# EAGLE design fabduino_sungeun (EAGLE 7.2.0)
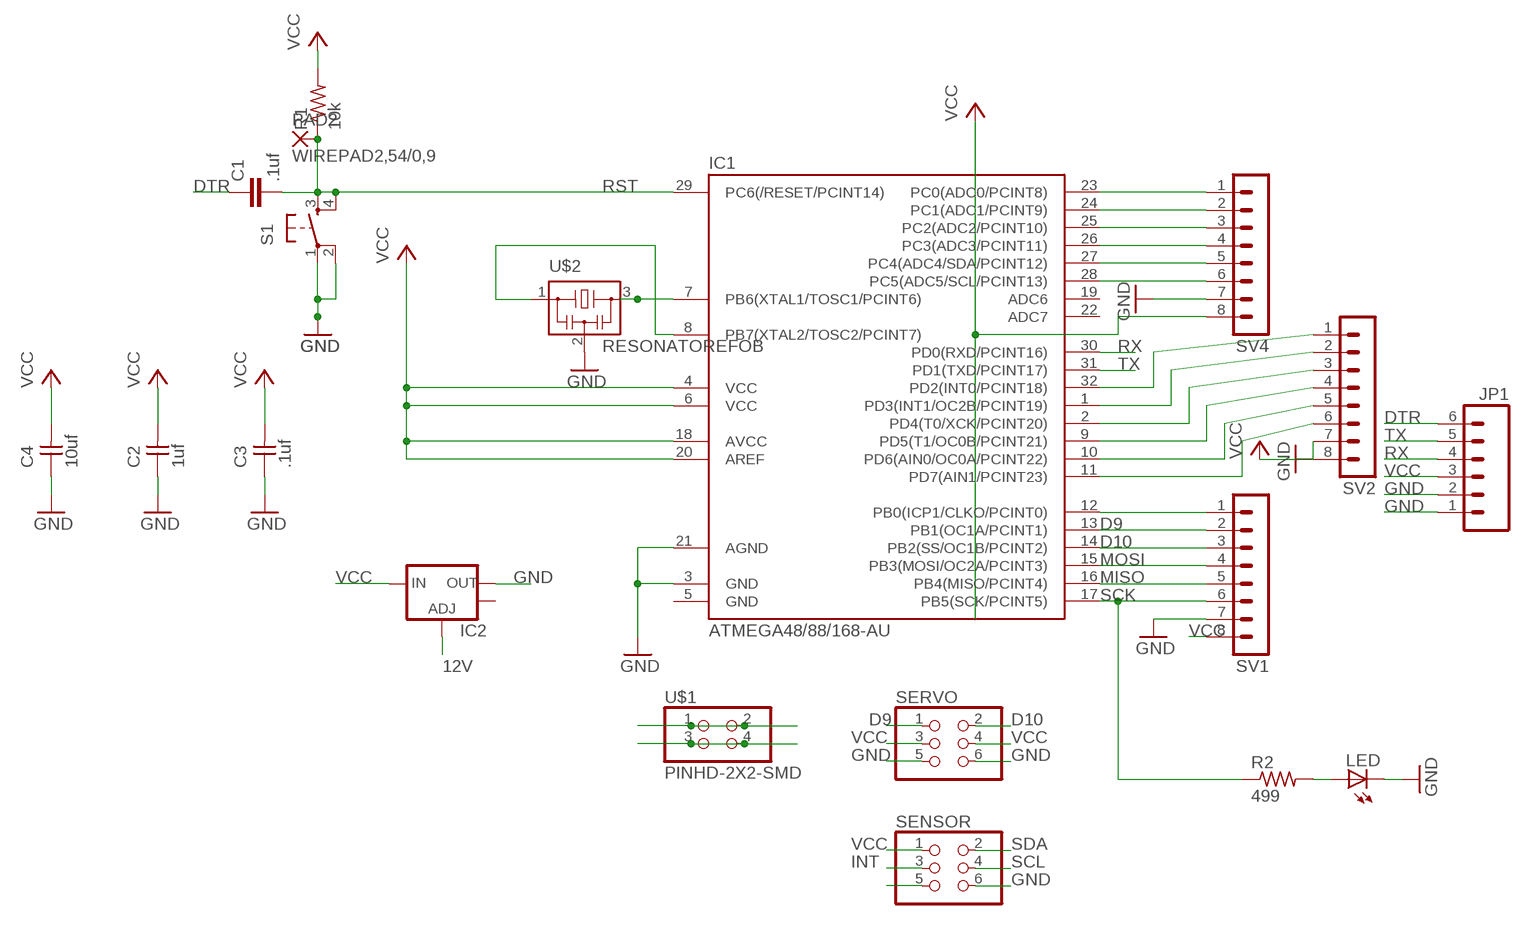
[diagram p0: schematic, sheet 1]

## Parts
C1  .1uf  C-EUC1206  [C1206]
C2  1uf  UNPOLARIZED_CAPACITOR1206  [1206]
C3  .1uf  UNPOLARIZED_CAPACITOR1206  [1206]
C4  10uf  UNPOLARIZED_CAPACITOR1206  [1206]
IC1  ATMEGA48/88/168-AU  [TQFP32-08]
IC2  V_REG_LM1117SOT223  [SOT223]
JP1  M06SMD  [1X06-SMD]
LED  LED1206  [1206]
PAD2  WIREPAD2,54/0,9  [2,54/0,9]
R1  10k  RESISTOR1206  [1206]
R2  499  RESISTOR1206  [1206]
S1  6MM_SWITCH6MM_SWITCH  [6MM_SWITCH]
SENSOR  PINHD-2X3-SMD  [2X03SMD]
SERVO  PINHD-2X3-SMD  [2X03SMD]
SV1  MA08-1  [MA08-1]
SV2  MA08-1  [MA08-1]
SV4  MA08-1  [MA08-1]
U$1  PINHD-2X2-SMD  [2X02SMD]
U$2  RESONATOREFOB  [EFOBM]

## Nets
12V: IC2.1(ADJ) U$1.1 U$1.2
D9: IC1.13(PB1(OC1A/PCINT1)) SERVO.1 SV1.2
D10: IC1.14(PB2(SS/OC1B/PCINT2)) SERVO.2 SV1.3
DTR: C1.1 JP1.6
GND: C2.1 C3.1 C4.1 IC1.3(GND) IC1.21(AGND) IC2.2(OUT) JP1.1 JP1.2 LED.2(C) S1.1(P) S1.2(P1) SENSOR.6 SERVO.5 SERVO.6 SV1.7 SV2.7 SV4.7 U$1.3 U$1.4 U$2.2
INT: IC1.32(PD2(INT0/PCINT18)) SENSOR.3 SV2.1
MISO: IC1.16(PB4(MISO/PCINT4)) SV1.5
MOSI: IC1.15(PB3(MOSI/OC2A/PCINT3)) SV1.4
N$1: IC1.8(PB7(XTAL2/TOSC2/PCINT7)) U$2.1
N$2: IC1.12(PB0(ICP1/CLKO/PCINT0)) SV1.1
N$3: IC1.23(PC0(ADC0/PCINT8)) SV4.1
N$4: IC1.24(PC1(ADC1/PCINT9)) SV4.2
N$5: IC1.25(PC2(ADC2/PCINT10)) SV4.3
N$6: IC1.26(PC3(ADC3/PCINT11)) SV4.4
N$9: IC1.7(PB6(XTAL1/TOSC1/PCINT6)) U$2.3
N$11: IC1.1(PD3(INT1/OC2B/PCINT19)) SV2.2
N$12: IC1.2(PD4(T0/XCK/PCINT20)) SV2.3
N$13: IC1.9(PD5(T1/OC0B/PCINT21)) SV2.4
N$14: IC1.10(PD6(AIN0/OC0A/PCINT22)) SV2.5
N$15: IC1.11(PD7(AIN1/PCINT23)) SV2.6
N$23: LED.1(A) R2.2
N$30: SENSOR.5
RST: C1.2 IC1.29(PC6(/RESET/PCINT14)) PAD2.1(P) R1.1 S1.3(S) S1.4(S1)
RX: IC1.30(PD0(RXD/PCINT16)) JP1.4
SCK: IC1.17(PB5(SCK/PCINT5)) R2.1 SV1.6
SCL: IC1.28(PC5(ADC5/SCL/PCINT13)) SENSOR.4 SV4.6
SDA: IC1.27(PC4(ADC4/SDA/PCINT12)) SENSOR.2 SV4.5
TX: IC1.31(PD1(TXD/PCINT17)) JP1.5
VCC: C2.2 C3.2 C4.2 IC1.4(VCC) IC1.6(VCC) IC1.18(AVCC) IC1.20(AREF) IC2.3(IN) JP1.3 R1.2 SENSOR.1 SERVO.3 SERVO.4 SV1.8 SV2.8 SV4.8
Unconnected: IC1.19(ADC6) IC1.22(ADC7) IC2.4(OUT)

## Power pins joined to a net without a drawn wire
GND: IC1.5(GND)

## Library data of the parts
C1 = rcl:C-EU: CAPACITOR, European symbol
C2-C4 = ng:UNPOLARIZED_CAPACITOR: unpolarized_capacitor
IC1 = atmega8:ATMEGA48/88/168
IC2 = SparkFun-PowerIC:V_REG_LM1117: Voltage Regulator LM1117 Standard adjustable voltage regulator but in SMD form. Spark Fun Electronics SKU : COM-00595; PROD_ID: VREG-08170
JP1 = SparkFun:M06: Header 6 Standard 6-pin 0.1" header. Use with straight break away headers (SKU : PRT-00116), right angle break away headers (PRT-00553), swiss pins (PRT-00743), machine pins (PRT-00117), and female headers (PRT-00115). Molex polarized connector foot print use with SKU : PRT-08094 with associated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
LED = ng:LED
PAD2 = wirepad:WIREPAD: Wire PAD connect wire on PCB
R1 R2 = ng:RESISTOR
S1 = ng:6MM_SWITCH: OMRON SWITCH
SENSOR SERVO = fab:PINHD-2X3-SMD: PIN HEADER
SV1 SV2 SV4 = con-lstb:MA08-1: PIN HEADER
U$1 = fab:PINHD-2X2-SMD
U$2 = fab:RESONATOR

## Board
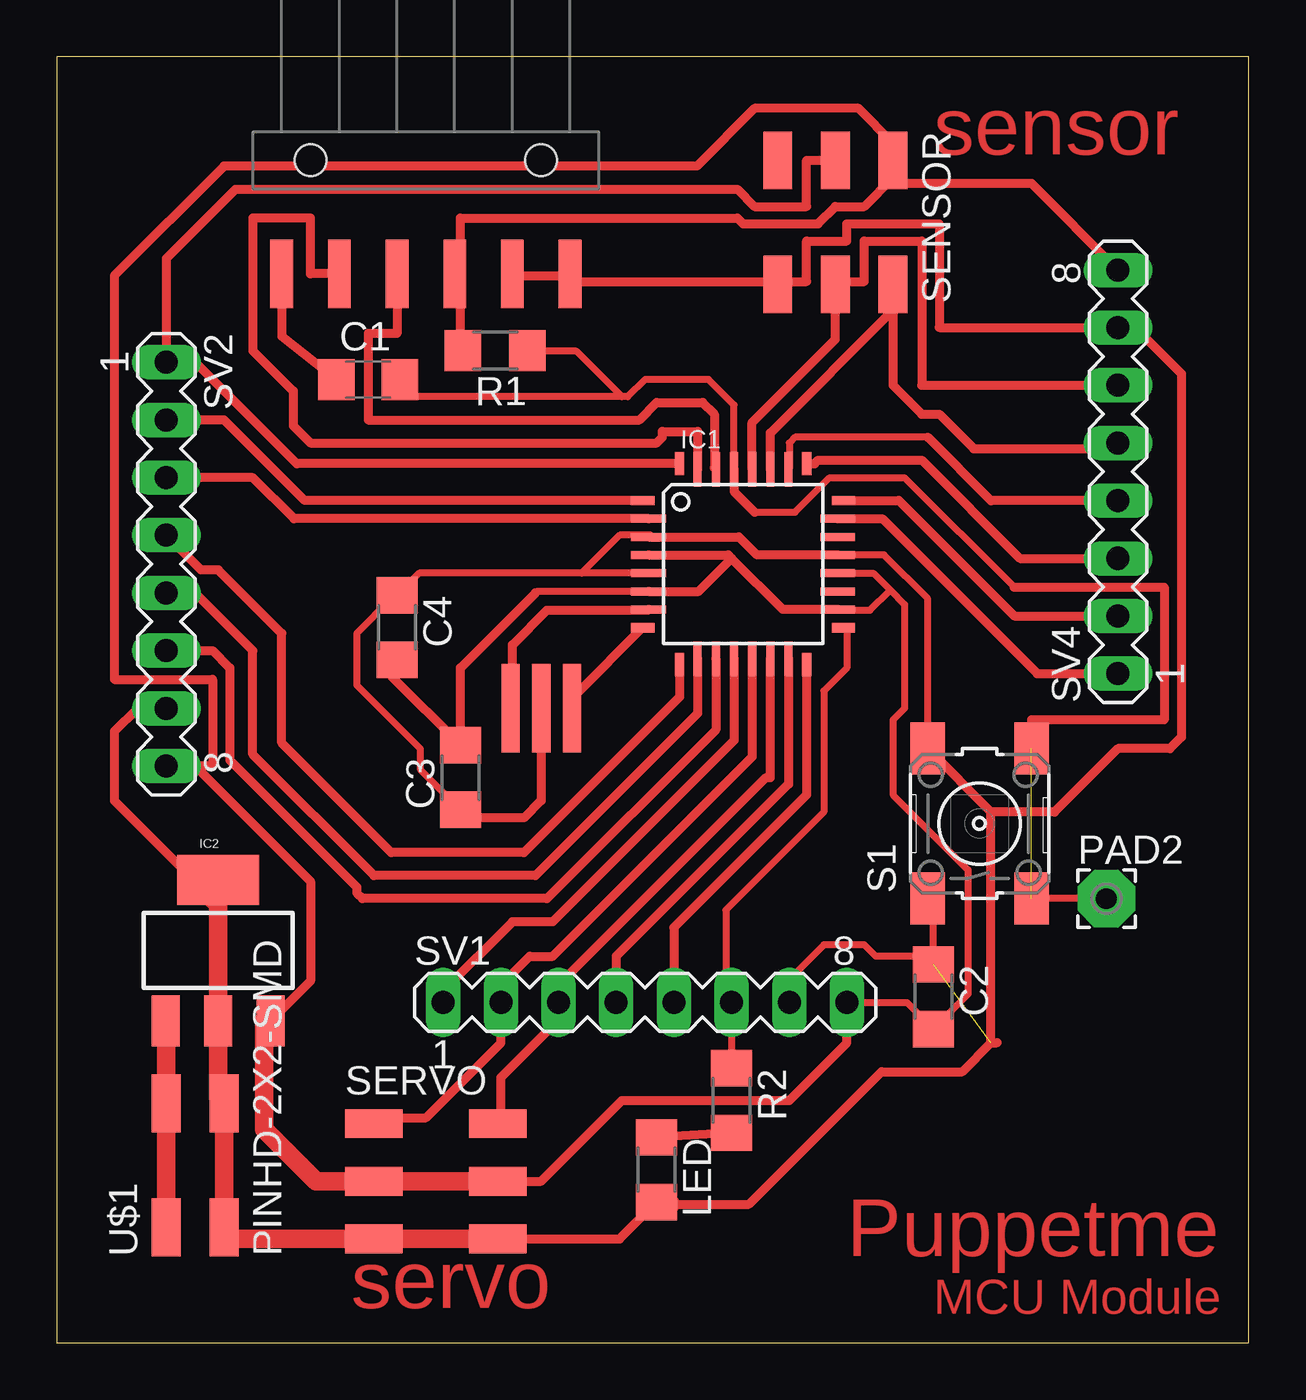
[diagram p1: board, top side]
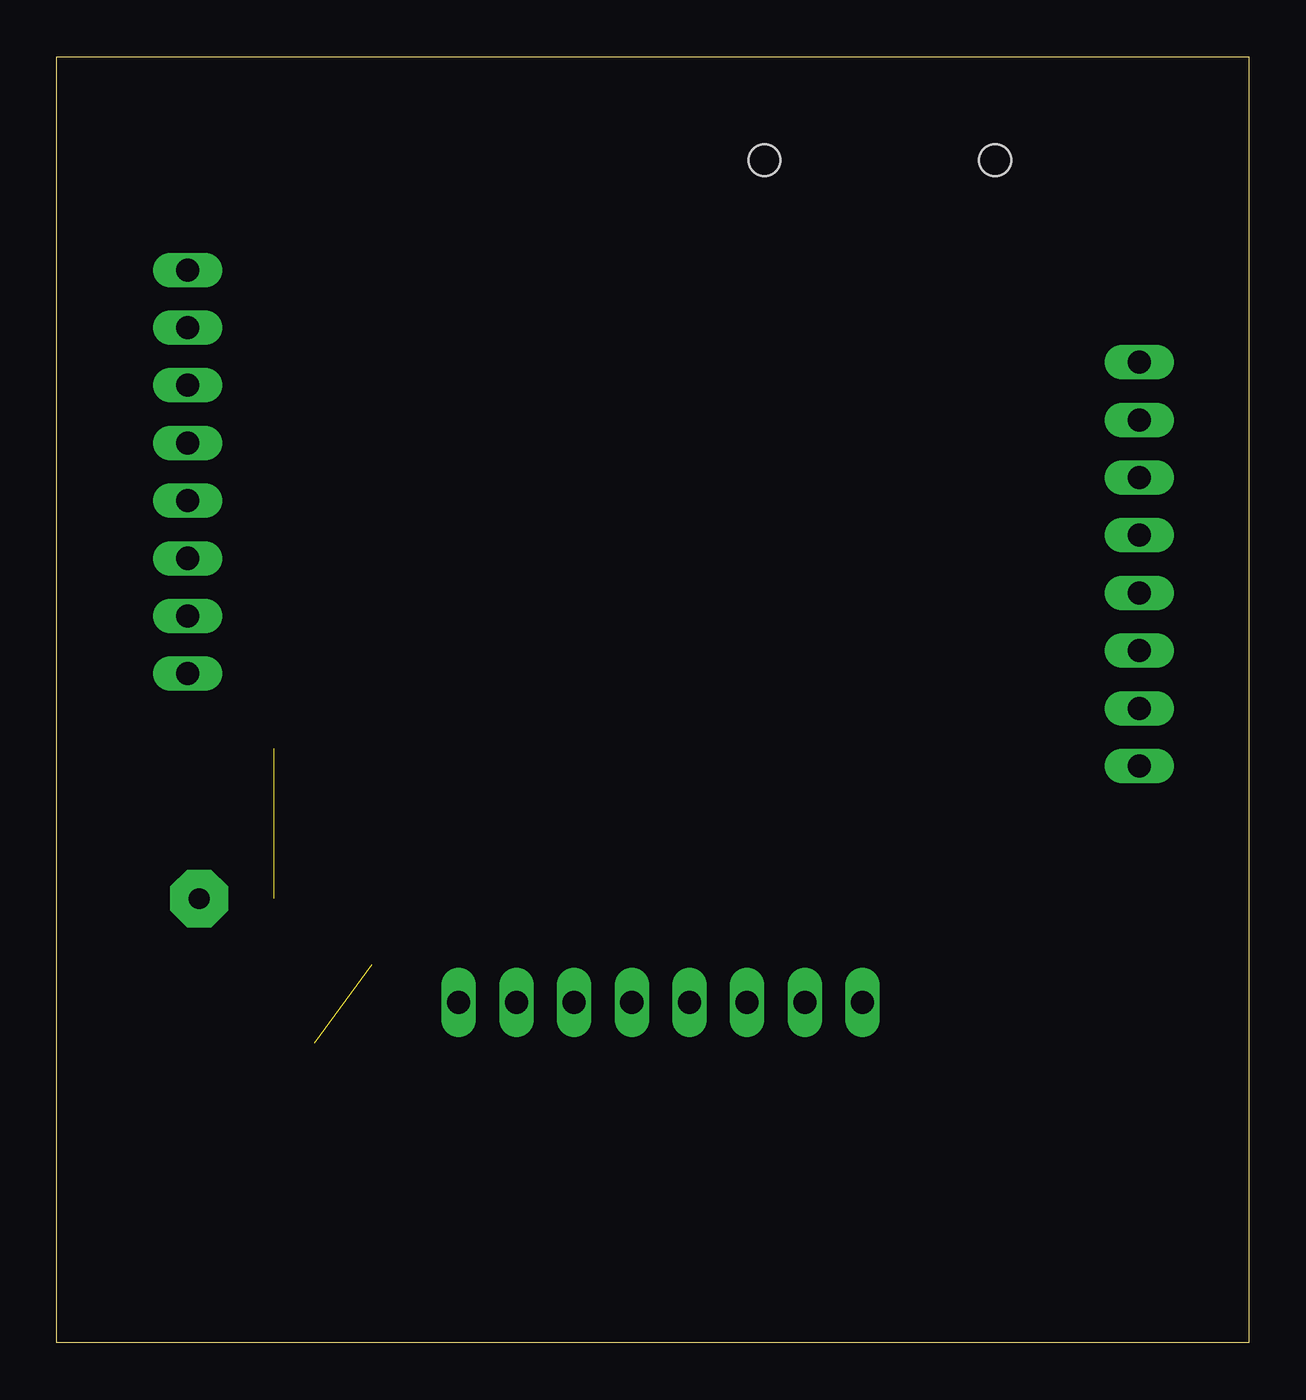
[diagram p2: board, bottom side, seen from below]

Size 52.5 x 56.63 mm. Coordinates in mm from the lower left corner, seen from the top.
Outline: 0,0 52.5,0 52.5,56.63 0,56.63 0,0
Copper layers (1*16): Top 0.035mm / dielectric 1.5mm / Bottom 0.035mm
Design rules "default": minimum track width 10mil, minimum drill 24mil, track to track 8mil, track to pad 8mil, pad to pad 8mil, via to via 8mil, smd to smd 8mil, copper to edge 40mil, drill to drill 8mil, minimum pad ring 10mil, minimum via ring 8mil, stop-mask expansion 4mil, vias tented up to drill 0mil, thermal gap 10mil

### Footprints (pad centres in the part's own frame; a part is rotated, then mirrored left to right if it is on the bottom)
C1206 = smd 1.6 x 1.8: 1 -1.4,0; 2 1.4,0
1206 = smd 1.6 x 1.803: 1 -1.422,0; 2 1.422,0
TQFP32-08 = smd 1.016 x 0.406: 1 -4.42,2.8; 8 -4.42,-2.8; 17 4.42,-2.8; 24 4.42,2.8 | smd 1.524 x 0.356: 2 -4.166,2; 3 -4.166,1.2; 4 -4.166,0.4; 5 -4.166,-0.4; 6 -4.166,-1.2; 7 -4.166,-2; 18 4.166,-2; 19 4.166,-1.2; 20 4.166,-0.4; 21 4.166,0.4; 22 4.166,1.2; 23 4.166,2 | smd 0.406 x 1.016: 9 -2.8,-4.42; 16 2.8,-4.42; 25 2.8,4.42; 32 -2.8,4.42 | smd 0.356 x 1.524: 10 -2,-4.166; 11 -1.2,-4.166; 12 -0.4,-4.166; 13 0.4,-4.166; 14 1.2,-4.166; 15 2,-4.166; 26 2,4.166; 27 1.2,4.166; 28 0.4,4.166; 29 -0.4,4.166; 30 -1.2,4.166; 31 -2,4.166
SOT223 = smd 1.219 x 2.235: 1 -2.311,-3.099; 2 0,-3.099; 3 2.311,-3.099 | smd 3.6 x 2.2: 4 0,3.099
1X06-SMD = smd 1 x 3: 1 -6.35,5; 2 -3.81,5; 3 -1.27,5; 4 1.27,5; 5 3.81,5; 6 6.35,5 | hole 1.4: -5.08,0; 5.08,0
2,54/0,9 = drill 0.914 pad 2.54 octagon: 1 0,0
6MM_SWITCH = smd 2.286 x 1.524: 1 -3.302,2.286; 2 3.302,2.286; 3 -3.302,-2.286; 4 3.302,-2.286
2X03SMD = smd 2.54 x 1.27: 1 -2.54,2.54; 2 2.92,2.54; 3 -2.54,0; 4 2.92,0; 5 -2.54,-2.54; 6 2.92,-2.54
MA08-1 = drill 1.016 long: 1 -8.89,0; 2 -6.35,0; 3 -3.81,0; 4 -1.27,0; 5 1.27,0; 6 3.81,0; 7 6.35,0; 8 8.89,0
2X02SMD = smd 2.54 x 1.27: 1 -2.54,1.27; 2 2.92,1.27; 3 -2.54,-1.27; 4 2.92,-1.27
EFOBM = smd 0.8 x 3.9: 1 -1.35,0; 2 0,0; 3 1.35,0

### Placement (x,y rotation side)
C1  13.72,42.42 0 top
C2  38.61,15.24 270 top
C3  17.78,24.89 90 top
C4  14.99,31.5 270 top
IC1  30.23,34.29 0 top
IC2  7.11,17.27 0 top
JP1  16.26,52.07 180 top
LED  26.42,7.62 270 top
PAD2  46.23,19.56 0 top
R1  19.3,43.69 180 top
R2  29.72,10.67 270 top
S1  40.64,22.86 90 top
SENSOR  34.29,49.53 270 top
SERVO  16.51,7.11 0 top
SV1  25.91,14.99 0 top
SV2  4.83,34.29 270 top
SV4  46.74,38.35 90 top
U$1  6.1,7.62 90 top
U$2  21.34,27.94 180 top

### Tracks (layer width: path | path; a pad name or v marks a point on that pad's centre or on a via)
12V
  Top 0.406: IC2.1 4.88,14.17 5.08,13.97 4.83,13.72 4.83,14.22
  Top 0.813: U$1.1 4.83,10.16 U$1.2 4.83,14.15 IC2.1
D9
  Top 0.406: IC1.13 30.63,25.8 21.84,17.02 20.83,17.02 19.56,15.75 SV1.2 19.56,13.21 16.26,9.91 14.22,9.91 SERVO.1
D10
  Top 0.406: IC1.14 31.43,24.89 31.24,24.89 22.1,15.75 SV1.3 22.1,14.22 19.56,11.68 19.56,9.65 SERVO.2
DTR
  Top 0.406: JP1.6 9.91,44.32 C1.1
GND  (1 unrouted)
  Top 0.305: S1.2 38.35,32.77 36.43,34.69 IC1.21 | IC1.5 23.11,33.89 | 23.11,33.89 15.96,33.89 C4.1 14.99,32.77 14.73,32.77 13.21,31.24 13.21,28.96 16,26.16 16,25.25 C3.1 | IC1.3 26.09,35.49 26.16,35.56 24.78,35.56 23.11,33.89 | S1.1 38.61,19.3 C2.1 38.61,16.76 38.35,17.02 36.07,17.02 35.56,17.53 33.78,17.53 32.26,16 SV1.7 | LED.2 26.42,6.1
  Top 0.406: IC1.3 30.04,35.49 30.84,34.69 IC1.21 | 7.87,4.57 U$1.3 | U$2.2 21.34,23.88 20.57,23.11 18.14,23.11 C3.1 | 41.15,13.21 39.88,11.94 36.32,11.94 30.48,6.1 26.92,6.1 | 41.15,13.21 41.15,23.37 | 41.15,23.37 S1.2 | JP1.2 20.24,47.07 20.32,46.99 22.53,46.99 JP1.1 22.61,46.99 22.86,46.74 31.62,46.74 SENSOR.6 32,46.61 32,46.74 33.02,46.74 33.02,48.51 34.8,48.51 34.8,49.28 38.86,49.28 38.86,44.7 SV4.7 47.5,44.7 49.53,42.67 49.53,26.67 49.02,26.16 46.74,26.16 43.94,23.37 41.15,23.37 | 41.15,13.21 41.4,13.21 | 5.08,27.94 SV2.7 3.56,27.94 2.54,26.92 2.54,23.88 6.73,19.69 | SERVO.6 24.79,4.57 LED.2
  Top 0.813: 6.73,19.69 7.11,19.3 IC2.2 7.11,10.79 U$1.4 U$1.3 | 7.87,4.57 SERVO.5 SERVO.6
  Top 1.016: 26.42,6.1 26.92,6.1
INT
  Top 0.406: IC1.32 10.57,38.71 6.1,43.18 SV2.1 4.83,47.75 7.87,50.8 29.97,50.8 30.73,50.04 33.02,50.04 33.02,52.07 SENSOR.3 34.04,51.82
MISO
  Top 0.406: IC1.16 33.02,24.13 27.18,18.29 SV1.5
MOSI
  Top 0.406: IC1.15 32.23,24.61 24.64,17.02 SV1.4
N$1
  Top 0.406: U$2.1 22.69,28.02 22.86,28.19 22.86,28.54 IC1.8
N$2
  Top 0.406: IC1.12 29.83,26.52 21.84,18.54 20.07,18.54 17.02,15.49 SV1.1
  Bottom 0.406: SV1.1 17.02,15.49
N$3
  Top 0.406: IC1.23 36.35,36.29 43.18,29.46 SV4.1
N$4
  Top 0.406: IC1.24 37.08,37.09 42.16,32 SV4.2
N$5
  Top 0.406: IC1.25 33.38,38.71 33.53,38.86 38.1,38.86 42.42,34.54 SV4.3
N$6
  Top 0.305: 38.35,39.88 32.51,39.88 32.26,39.62 32.26,38.49 IC1.26
  Top 0.406: SV4.4 41.15,37.08 38.35,39.88
N$9
  Top 0.406: U$2.3 20.07,27.94 20.07,30.73 21.59,32.26 26.03,32.26 IC1.7
N$11
  Top 0.406: IC1.1 10.92,37.09 7.37,40.64 SV2.2
N$12
  Top 0.406: IC1.2 10.45,36.29 8.64,38.1 SV2.3
N$13
  Top 0.406: IC1.9 27.43,28.44 20.57,21.59 14.73,21.59 9.91,26.42 9.91,31.24 7.11,34.04 6.35,34.04 SV2.4
N$14
  Top 0.406: IC1.10 28.23,27.72 21.08,20.57 13.97,20.57 8.64,25.91 8.64,30.48 6.1,33.02 SV2.5
N$15
  Top 0.406: IC1.11 29.03,26.99 21.59,19.56 13.46,19.56 13.21,19.81 13.21,20.07 7.62,25.65 7.62,29.72 6.86,30.48 SV2.6
N$23
  Top 0.406: R2.2 LED.1
RST  (1 unrouted)
  Top 0.305: IC1.29 29.83,41.29 28.7,42.42 25.91,42.42 25.15,41.66 24.89,41.66 | 24.89,41.66 15.88,41.66 C1.2 | PAD2.1 S1.3 | R1.1 22.86,43.69 24.89,41.66 | 30.73,36.58 32.51,36.58 34.04,38.1 37.34,38.1 42.16,33.27
  Top 0.406: IC1.29 29.83,37.48 30.73,36.58 | 42.16,33.27 48.77,33.27 48.77,27.43 42.93,27.43 S1.4
RX
  Top 0.406: JP1.4 14.99,44.45 13.72,44.45 13.72,40.64 25.65,40.64 26.42,41.4 28.45,41.4 28.96,40.89 28.96,38.53 IC1.30
SCK
  Top 0.305: IC1.17 34.79,31.49 34.8,31.5 34.8,29.72 33.78,28.7 33.78,23.37 29.46,19.05 29.46,15.24 SV1.6 R2.1
SCL
  Top 0.406: IC1.28 30.63,40.53 34.29,44.2 SENSOR.4 34.29,46.74 35.56,46.74 35.56,48.51 38.1,48.51 38.1,42.16 SV4.6
SDA
  Top 0.406: IC1.27 31.43,40.06 36.83,45.47 SENSOR.2 36.83,42.16 38.1,40.89 38.86,40.89 40.39,39.37 46.48,39.37 SV4.5
TX
  Top 0.406: JP1.5 11.18,47.07 11.18,49.53 8.64,49.53 8.64,43.69 10.41,41.91 10.41,40.39 11.18,39.62 26.42,39.62 26.67,39.88 26.67,40.13 28.23,40.13 IC1.31
VCC
  Top 0.305: JP1.3 17.7,47.07 17.78,46.99 17.78,43.79 R1.2 | IC1.20 35.96,33.89 36.7,33.15 | 36.7,33.15 37.34,32.51 37.34,27.94 36.83,27.43 36.83,24.13 40.13,20.83 40.13,15.34 C2.2 | IC1.18 34.77,32.29 34.8,32.26 35.81,32.26 36.7,33.15 | IC1.6 21.15,33.09 21.08,33.02 | C2.2 38.61,13.72 38.35,13.46 37.85,13.46 | SV1.8 37.44,14.99 C2.2
  Top 0.406: IC1.18 31.97,32.29 29.72,34.54 | 29.72,34.54 29.57,34.69 IC1.4 | IC1.6 28.26,33.09 29.72,34.54 | 9.14,14.22 9.19,14.17 IC2.3 11.18,15.93 11.18,20.32 6.1,25.4 SV2.8 6.86,25.4 6.86,29.21 2.54,29.21 2.54,46.99 7.37,51.82 28.19,51.82 30.73,54.36 35.31,54.36 36.83,52.83 SENSOR.1 | C4.2 14.83,30.07 14.73,29.97 14.73,29.36 C3.2 17.78,29.72 21.08,33.02 | 36.83,51.31 36.83,51.05 42.93,51.05 SV4.8 | 36.83,51.31 SENSOR.1 | 37.08,51.82 SENSOR.1 | R1.2 17.78,43.69 17.78,49.53 29.97,49.53 30.23,49.28 33.53,49.28 34.29,50.04 35.56,50.04 36.83,51.31 | SERVO.4 21.34,7.11 24.89,10.67 32.26,10.67 34.8,13.21 SV1.8
  Top 0.813: 9.14,14.22 9.14,9.4 11.43,7.11 SERVO.3 SERVO.4

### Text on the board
Top: sensor | Puppetme | servo | MCU Module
